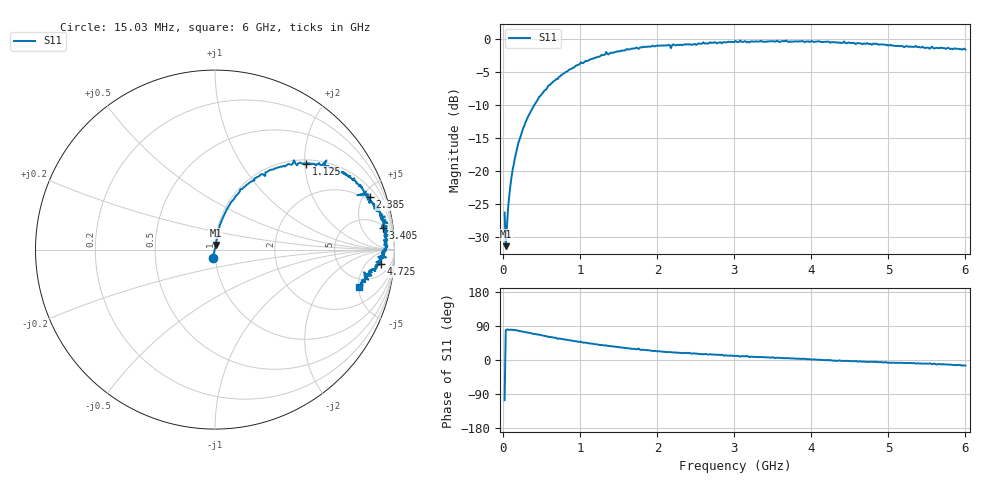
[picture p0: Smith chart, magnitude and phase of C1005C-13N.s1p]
!	Network	Analyzer	HP8753E.07.74:	Oct	30	2002	Serial	No.	JP38451487
!	Hewlett-Packard
!	7	Sep	2009	8:44:59
!	Frequency	S11
#	HZ	S	RI	R	50
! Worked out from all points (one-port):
!   400 points, 15.03 MHz to 6 GHz, reference 50 ohm
!   lowest |S11| = -31.4 dB at 30.03 MHz (marker M1), VSWR 1.06, Z = 50.5 + j2.68 ohm
!   |S11| at or under -10 dB: start of sweep to 401.9 MHz
!   S11 on the Smith chart (normalised r, x): 15.03 MHz: 0.97, -0.09; 1.125 GHz: 1.09, +2.02; 2.385 GHz: 1.65, +5.60; 3.405 GHz: 6, +13; 4.725 GHz: 11, -13; 6 GHz: 3.75, -5.04
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1.502992e7  -0.0133 -0.0467
3.002985e7  0.00536 0.0265
6.00297e7  0.00877 0.0518
1.050295e8  0.0157 0.0888
1.650292e8  0.0263 0.136
2.550287e8  0.0555 0.203
4.650277e8  0.142 0.337
7.650262e8  0.304 0.442
1.005025e9  0.44 0.498
1.125024e9  0.506 0.479
1.335023e9  0.621 0.497
1.515022e9  0.672 0.44
1.725021e9  0.754 0.41
1.755021e9  0.722 0.426
1.785021e9  0.771 0.386
1.93502e9  0.812 0.358
2.145019e9  0.841 0.323
2.175019e9  0.793 0.303
2.205019e9  0.854 0.308
2.265019e9  0.851 0.299
2.385018e9  0.862 0.292
3.015015e9  0.946 0.184
3.405013e9  0.937 0.119
3.765011e9  0.947 0.0728
4.515007e9  0.93 -0.0438
4.725006e9  0.925 -0.08
5.265004e9  0.865 -0.122
6e9  0.802 -0.21
